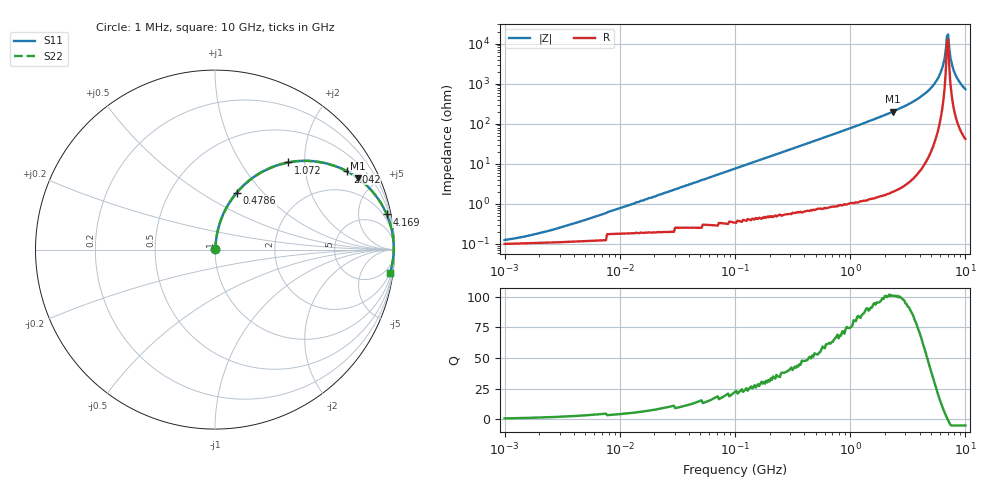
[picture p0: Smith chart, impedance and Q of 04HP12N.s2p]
# MHz S MA R 50
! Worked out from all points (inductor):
!   401 points, 1 MHz to 10 GHz, reference 50 ohm
!   read as one part in series: L = 12 nH near 4.677 MHz
!   highest Q = 101 at 2.344 GHz (marker M1), where L = 13.5 nH
!   self-resonance near 6.918 GHz
!   S11 on the Smith chart (normalised r, x): 1 MHz: 1.00, +0.00; 478.6 MHz: 1.01, +0.73; 1.072 GHz: 1.02, +1.66; 2.042 GHz: 1.03, +3.37; 4.169 GHz: 1.13, +9.73; 10 GHz: 2, -15
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1  0.001238 37.4  0.999 -0.0  0.999 -0.0  0.001238 37.4
2.042  0.001893 54.2  0.999 -0.1  0.999 -0.1  0.001893 54.2
4.677  0.003759 69.4  0.999 -0.2  0.999 -0.2  0.003759 69.4
21.878  0.017 82.0  0.998 -0.9  0.998 -0.9  0.017 82.0
102.329  0.077 83.0  0.994 -4.4  0.994 -4.4  0.077 83.0
467.735  0.332 69.5  0.937 -19.4  0.937 -19.4  0.332 69.5
478.63  0.339 69.1  0.934 -19.8  0.934 -19.8  0.339 69.1
1071.519  0.634 50.0  0.766 -39.3  0.766 -39.3  0.634 50.0
2041.738  0.856 30.6  0.509 -58.8  0.509 -58.8  0.856 30.6
2187.762  0.874 28.6  0.478 -60.9  0.478 -60.9  0.874 28.6
2344.229  0.89 26.6  0.447 -62.9  0.447 -62.9  0.89 26.6
4168.694  0.977 11.6  0.201 -77.5  0.201 -77.5  0.977 11.6
5128.614  0.99 6.8  0.119 -81.6  0.119 -81.6  0.99 6.8
5888.437  0.994 3.8  0.066 -83.1  0.066 -83.1  0.994 3.8
6309.573  0.995 2.3  0.04 -82.1  0.04 -82.1  0.995 2.3
6760.83  0.996 0.8  0.014 -71.9  0.014 -71.9  0.996 0.8
6918.31  0.996 0.3  0.006495 -47.8  0.006495 -47.8  0.996 0.3
7244.36  0.995 -0.7  0.013 69.0  0.013 69.0  0.995 -0.7
7585.776  0.995 -1.7  0.03 78.9  0.03 78.9  0.995 -1.7
8128.305  0.993 -3.2  0.056 81.2  0.056 81.2  0.993 -3.2
8912.509  0.99 -5.2  0.091 80.8  0.091 80.8  0.99 -5.2
10000  0.983 -7.8  0.135 79.0  0.135 79.0  0.983 -7.8
